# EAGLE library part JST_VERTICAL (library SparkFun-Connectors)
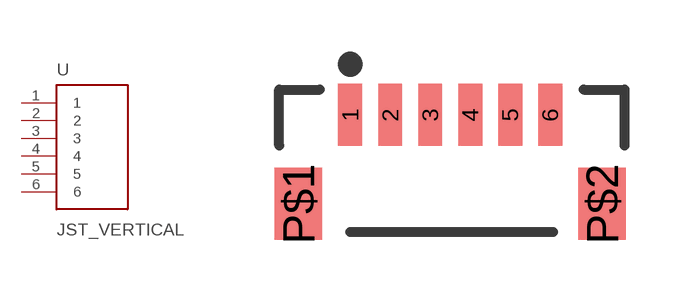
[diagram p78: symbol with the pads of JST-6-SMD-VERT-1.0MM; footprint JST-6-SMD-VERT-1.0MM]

Designator prefix -

## JST_VERTICAL (PROD_ID: CONN-08249)  [JST-6-SMD-VERT-1.0MM]
1  1
2  2
3  3
4  4
5  5
6  6

## Footprint JST-6-SMD-VERT-1.0MM (pad centres in mm)
smd 0.6 x 1.55: 1 -2.54,1.27; 2 -1.54,1.27; 3 -0.54,1.27; 4 0.46,1.27; 5 1.46,1.27; 6 2.46,1.27
smd 1.2 x 1.8: P$1 -3.84,-0.955; P$2 3.76,-0.955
